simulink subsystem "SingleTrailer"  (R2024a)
settings: Solver=VariableStepAuto  StartTime=0.0  StopTime=10.0  RelTol=1e-3
undefined symbols (not defined in the file): D, PlntTraCGHgtAxl, PlntTraDstCGMiddleAxl, PlntTraHtchCxy, PlntTraHtchCz, PlntTraHtchF0z, PlntTraHtchKxy, PlntTraHtchKz, PlntTraInitLatPos, PlntTraInitLatVel, PlntTraInitLongPos, PlntTraInitLongVel, PlntTraInitPitchAng, PlntTraInitPitchRate, PlntTraInitRollAng, PlntTraInitRollRate, PlntTraInitVertPos, PlntTraInitVertVel, PlntTraInitYawAng, PlntTraInitYawRate, PlntTraMass, PlntTraNumWhlFrntAxl, PlntTraPitchMomentInertia, PlntTraRollMomentInertia, PlntTraTrckWdth, PlntTraYawMomentInertia, repmat, Row, vector
libraries: autolibutils x7, sharedtransform x4, vehdynlibeom x2, vehdynlibsuspension x1, matrix_library x1
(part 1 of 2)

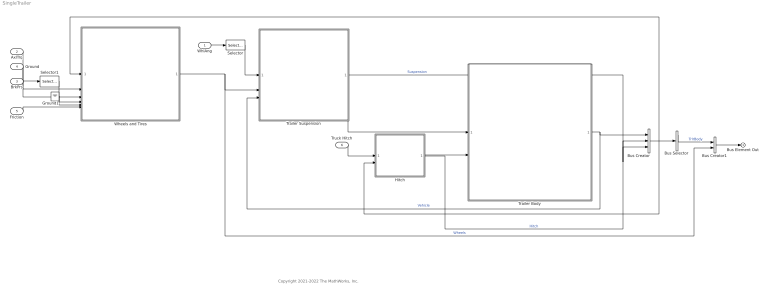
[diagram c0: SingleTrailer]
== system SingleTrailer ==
  note: Copyright 2021-2022 The MathWorks, Inc.
  WhlAng : Inport
  AxlTrq : Inport  Port=2
  BrkPrs : Inport  Port=3
  Ground : Inport  Port=4
  Friction : Inport  Port=5
  Truck Hitch : Inport  Port=6
  Bus Creator : BusCreator  Inputs=3
  Bus Creator1 : BusCreator  Inputs=2
  Bus Selector : BusSelector  OutputSignals=Vehicle.InertFrm,Vehicle.BdyFrm,Hitch,Suspension  OutputAsBus=on
  Ground1 : Ground
  Hitch : Subsystem  Variant=on  VariantControlMode=label  LabelModeActiveChoice=Hitch 3DOF
  Selector : Selector  IndexOptions=Index vector (dialog)  Indices=[1 2]  OutputSizes=1
  Selector1 : Selector  IndexOptions=Index vector (dialog)  Indices=[1 2]  OutputSizes=1
  Trailer Body : Subsystem  Variant=on  VariantControlMode=label  LabelModeActiveChoice=Trailer Body 3DOF
  Trailer Suspension : Subsystem
  Wheels and Tires : Subsystem  Variant=on  VariantControlMode=label  VariantControl=Choice  LabelModeActiveChoice=MF Tires Longitudinal and Lateral
  Bus Element Out : Outport
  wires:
  Trailer Suspension/1(SuspWheel) -> Bus Creator/2  "Suspension"
  Trailer Suspension/2(SuspChassis) -> Trailer Body/1(Suspension)
  Bus Selector/1 -> Bus Creator1/1  "TrlrBody"
  AxlTrq/1 -> Wheels and Tires/2(AxlTrq)
  Bus Creator/1 -> Bus Selector/1, Wheels and Tires/1(Suspension), Hitch/2(Trailer)
  Wheels and Tires/1(Wheels) -> Bus Creator1/2, Trailer Suspension/2(Wheels)  "Wheels"
  BrkPrs/1 -> Selector1/1
  WhlAng/1 -> Selector/1
  Friction/1 -> Wheels and Tires/6(Friction)
  Trailer Body/1(Vehicle) -> Bus Creator/1, Trailer Suspension/3(Veh)  "Vehicle"
  Truck Hitch/1 -> Hitch/1(Vehicle)
  Selector/1 -> Trailer Suspension/1(Steering)
  Selector1/1 -> Wheels and Tires/4(BrkPrs)
  Ground/1 -> Wheels and Tires/3(Ground Input)
  Ground1/1 -> Wheels and Tires/5(GndDCM)
  Hitch/1(Vehicle Hitch) -> Bus Creator/3  "Hitch"
  Hitch/2(Trailer Hitch) -> Trailer Body/2(Hitch)
  Bus Creator1/1 -> Bus Element Out/1

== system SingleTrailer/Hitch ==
  note: 1) Add Subsystem or Model blocks as valid variant choices. 2) You cannot connect blocks at this level. At simulation, connectivity is automatically determined, based on the active variant and port name matching.
  Vehicle : Inport
  Trailer : Inport  Port=2
  3DOF : Subsystem  VariantControl=Hitch 3DOF
  6DOF : Subsystem  VariantControl=Hitch 6DOF
  Vehicle Hitch : Outport
  Trailer Hitch : Outport  Port=2

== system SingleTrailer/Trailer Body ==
  note: 1) Add Subsystem or Model blocks as valid variant choices. 2) You cannot connect blocks at this level. At simulation, connectivity is automatically determined, based on the active variant and port name matching.
  Suspension : Inport
  Hitch : Inport  Port=2
  Trailer Body 3DOF : Subsystem  VariantControl=Trailer Body 3DOF
  Trailer Body 6DOF : Subsystem  VariantControl=Trailer Body 6DOF
  Vehicle : Outport

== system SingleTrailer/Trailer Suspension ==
  Steering : Inport
  Wheels : Inport  Port=2
  Veh : Inport  Port=3
  Bus Creator : BusCreator  Inputs=2
  Solid Axle Suspension : Subsystem  VariantControl=MacPherson Front Suspension Solid Axle Rear Suspension
  Susp2Wheel : Subsystem
  Wheel2Susp : Subsystem
  SuspWheel : Outport
  SuspChassis : Outport  Port=2
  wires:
  Steering/1 -> Solid Axle Suspension/1(Steer)
  Veh/1 -> Solid Axle Suspension/2(Vehicle), Wheel2Susp/1(Veh)
  Bus Creator/1 -> SuspChassis/1
  Wheels/1 -> Wheel2Susp/2(Wheels)
  Susp2Wheel/1(SuspWheel) -> Wheel2Susp/3(SuspWheel), Bus Creator/2, SuspWheel/1  "SuspWheel"
  Wheel2Susp/1(Wheels2Susp) -> Susp2Wheel/2(WheelSusp), Solid Axle Suspension/3(Wheels)
  Solid Axle Suspension/1(Suspension) -> Bus Creator/1, Susp2Wheel/1(Susp)  "SuspChassis"

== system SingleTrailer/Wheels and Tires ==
  Suspension : Inport
  AxlTrq : Inport  Port=2
  Ground Input : Inport  Port=3
  BrkPrs : Inport  Port=4
  GndDCM : Inport  Port=5
  Friction : Inport  Port=6
  Combined Slip Tires Longitudinal : Subsystem  VariantControl=Combined Slip Tires Longitudinal  ReferencedSubsystem=CombinedSlipTrailerTiresLongitudinal
  Fiala Tires Longitudinal and Lateral : Subsystem  VariantControl=Fiala Tires Longitudinal and Lateral  ReferencedSubsystem=FialaTrailerTires
  MF Tires Longitudinal : Subsystem  VariantControl=MF Tires Longitudinal  ReferencedSubsystem=MFTrailerTiresLongitudinal
  MF Tires Longitudinal and Lateral : Subsystem  VariantControl=MF Tires Longitudinal and Lateral  ReferencedSubsystem=MFTrailerTires
  Wheels : Outport

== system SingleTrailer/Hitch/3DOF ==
  Vehicle : Inport
  Trailer : Inport  Port=2
  Bus Selector : BusSelector  OutputSignals=Body.InertFrm.Hitch.Disp.X,Body.InertFrm.Hitch.Disp.Y,Body.InertFrm.Cg.Ang.psi,Body.InertFrm.Hitch.Vel.Xdot,Body.InertFrm.Hitch.Vel.Ydot
  Bus Selector1 : BusSelector  OutputSignals=Vehicle.InertFrm.HitchF.Disp.X,Vehicle.InertFrm.HitchF.Disp.Y,Vehicle.InertFrm.Cg.Ang.psi,Vehicle.BdyFrm.Forces.HitchF.Fz,Vehicle.InertFrm.HitchF.Vel.Xdot,Vehicle.InertFrm.HitchF.Vel.Ydot
  Mux : Mux  Inputs=6
  Mux1 : Mux  Inputs=6
  Subsystem3 : Subsystem
  Vehicle Hitch : Outport
  Trailer Hitch : Outport  Port=2
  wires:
  Subsystem3/9(Trailer FzOut) -> Mux/3
  Mux1/1 -> Vehicle Hitch/1
  Vehicle/1 -> Bus Selector/1
  Mux/1 -> Trailer Hitch/1
  Trailer/1 -> Bus Selector1/1
  Bus Selector/1 -> Subsystem3/1(Vehicle X)  "<X>"
  Bus Selector/2 -> Subsystem3/2(Vehicle Y)  "<Y>"
  Bus Selector/3 -> Subsystem3/3(Vehicle psi)  "<psi>"
  Bus Selector1/1 -> Subsystem3/6(Trailer X)  "<X>"
  Bus Selector1/2 -> Subsystem3/7(Trailer Y)  "<Y>"
  Bus Selector1/4 -> Subsystem3/9(Trailer Fz)  "<Fz>"
  Bus Selector1/3 -> Subsystem3/8(Trailer psi)  "<psi>"
  Subsystem3/1(Vehicle Fx) -> Mux1/1
  Subsystem3/2(Vehicle Fy) -> Mux1/2
  Subsystem3/3(Vehicle Fz) -> Mux1/3
  Subsystem3/7(Trailer Fx) -> Mux/1
  Subsystem3/8(Trailer Fy) -> Mux/2
  Bus Selector/4 -> Subsystem3/4(Vehicle Xdot)  "<Xdot>"
  Bus Selector/5 -> Subsystem3/5(Vehicle Ydot)  "<Ydot>"
  Bus Selector1/5 -> Subsystem3/10(Trailer Xdot)  "<Xdot>"
  Bus Selector1/6 -> Subsystem3/11(Trailer Ydot)  "<Ydot>"
  Subsystem3/10(Trailer Mhx) -> Mux/4
  Subsystem3/11(Trailer Mhy) -> Mux/5
  Subsystem3/12(Trailer Mhz) -> Mux/6
  Subsystem3/4(Vehicle Mhx) -> Mux1/4
  Subsystem3/5(Vehicle Mhy) -> Mux1/5
  Subsystem3/6(Vehicle Mhz) -> Mux1/6

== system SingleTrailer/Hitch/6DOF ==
  Vehicle : Inport
  Trailer : Inport  Port=2
  Bus Selector : BusSelector  OutputSignals=InertFrm.Hitch.Disp.X,InertFrm.Hitch.Disp.Y,InertFrm.Hitch.Disp.Z,InertFrm.Hitch.Vel.Xdot,InertFrm.Hitch.Vel.Ydot,InertFrm.Hitch.Vel.Zdot,InertFrm.Cg.Ang.psi
  Bus Selector1 : BusSelector  OutputSignals=Vehicle.InertFrm.HitchF.Disp.X,Vehicle.InertFrm.HitchF.Disp.Y,Vehicle.InertFrm.HitchF.Disp.Z,Vehicle.InertFrm.HitchF.Vel.Xdot,Vehicle.InertFrm.HitchF.Vel.Ydot,Vehicle.InertFrm.HitchF.Vel.Zdot,Vehicle.InertFrm.Cg.Ang.psi
  Mux : Mux  Inputs=6
  Mux1 : Mux  Inputs=6
  Subsystem3 : Subsystem
  Vehicle Hitch : Outport
  Trailer Hitch : Outport  Port=2
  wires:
  Subsystem3/9(Trailer Fz) -> Mux/3
  Mux1/1 -> Vehicle Hitch/1
  Vehicle/1 -> Bus Selector/1
  Mux/1 -> Trailer Hitch/1
  Trailer/1 -> Bus Selector1/1
  Bus Selector/1 -> Subsystem3/1(Vehicle X)  "<X>"
  Bus Selector/2 -> Subsystem3/2(Vehicle Y)  "<Y>"
  Bus Selector/7 -> Subsystem3/7(Vehicle psi)  "<psi>"
  Bus Selector1/1 -> Subsystem3/8(Trailer X)  "<X>"
  Bus Selector1/2 -> Subsystem3/9(Trailer Y)  "<Y>"
  Bus Selector1/7 -> Subsystem3/14(Trailer psi)  "<psi>"
  Subsystem3/1(Vehicle Fx) -> Mux1/1
  Subsystem3/2(Vehicle Fy) -> Mux1/2
  Subsystem3/3(Vehicle Fz) -> Mux1/3
  Subsystem3/7(Trailer Fx) -> Mux/1
  Subsystem3/8(Trailer Fy) -> Mux/2
  Bus Selector1/3 -> Subsystem3/10(Trailer Z)  "<Z>"
  Bus Selector/3 -> Subsystem3/3(Vehicle Z)  "<Z>"
  Bus Selector/6 -> Subsystem3/6(Vehicle Zdot)  "<Zdot>"
  Bus Selector1/6 -> Subsystem3/13(Trailer Zdot)  "<Zdot>"
  Bus Selector1/5 -> Subsystem3/12(Trailer Ydot)  "<Ydot>"
  Bus Selector1/4 -> Subsystem3/11(Trailer Xdot)  "<Xdot>"
  Bus Selector/4 -> Subsystem3/4(Vehicle Xdot)  "<Xdot>"
  Bus Selector/5 -> Subsystem3/5(Vehicle Ydot)  "<Ydot>"
  Subsystem3/10(Trailer Mhx) -> Mux/4
  Subsystem3/11(Trailer Mhy) -> Mux/5
  Subsystem3/12(Trailer Mhz) -> Mux/6
  Subsystem3/4(Vehicle Mhx) -> Mux1/4
  Subsystem3/5(Vehicle Mhy) -> Mux1/5
  Subsystem3/6(Vehicle Mhz) -> Mux1/6

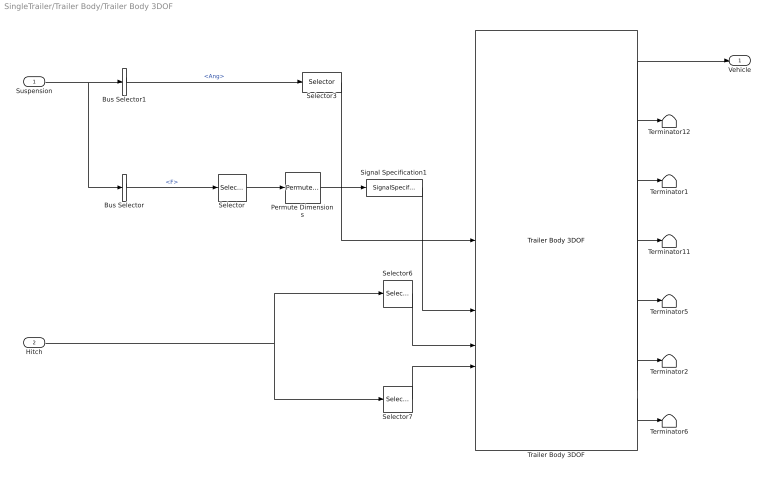
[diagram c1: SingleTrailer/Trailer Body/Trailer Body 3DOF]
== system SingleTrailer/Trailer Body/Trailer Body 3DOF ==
  Suspension : Inport
  Hitch : Inport  Port=2
  Bus Selector : BusSelector  OutputSignals=SuspChassis.Veh.F
  Bus Selector1 : BusSelector  OutputSignals=SuspChassis.Whl.Ang
  Permute Dimensions : PermuteDimensions
  Selector : Selector  NumberOfDimensions=2  InputPortWidth=3  IndexOptions=Index vector (dialog),Index vector (dialog)  Indices=[1 2],[1 2]  OutputSizes=1,1
  Selector3 : Selector  NumberOfDimensions=2  InputPortWidth=6  IndexOptions=Index vector (dialog),Index vector (dialog)  Indices=3,[1 2]  OutputSizes=1,1
  Selector6 : Selector  InputPortWidth=6  IndexOptions=Index vector (dialog)  Indices=[1 2 3]  OutputSizes=1
  Selector7 : Selector  InputPortWidth=6  IndexOptions=Index vector (dialog)  Indices=[4 5 6]  OutputSizes=1
  Signal Specification1 : SignalSpecification  Unit=N
  Terminator{1..2,5..6,11..12} (6 alike) : Terminator
  Trailer Body 3DOF : vehdynlibeom/Trailer Body 3DOF  trackMode=Dual 1-axle  inputMode=External forces  frontSteerMode=on  middleSteerMode=off  rearSteerMode=off  windMode=off  muMode=off  extFMode=off  extMMode=off  FhtchFMode=on  FhtchMMode=on  RhtchFMode=off  RhtchMMode=off  extXo=off  extpsio=off  extxdoto=off  extro=off  extYo=off  extTamb=off  extydoto=off  aMode=2  NF=PlntTraNumWhlFrntAxl  NM=PlntTraNumWhlMiddleAxl  NR=PlntTraNumWhlRearAxl  m=PlntTraMass  a=PlntTraDstCGFrntAxl  b=PlntTraDstCGMiddleAxl  c=PlntTraDstCGRearAxl  h=PlntTraCGHgtAxl  dh_f=PlntTraHtchDstFrnt  hh_f=PlntTraHtchHgtAxlFrnt  dh_r=7.5  hh_r=0.6  X_o=PlntTraInitLongPos  xdot_o=PlntTraInitLongVel  Lcpm=2.75  CalphaMode=off  sigmaMode=on  d=0  hl_f=0  hl_r=0  w_f=PlntTraTrckWdth  w_m=PlntTraTrckWdth  w_r=PlntTraTrckWdth  Cy_f=12e3  Cy_m=11e3  Cy_r=11e3  sigma_f=.1  sigma_m=.1  sigma_r=.1  alpha_f_brk=[-.1 .1]  Cy_f_data=[-9e3 9e3]  alpha_m_brk=[-.1 .1]  Cy_m_data=[-9e3 9e3]  alpha_r_brk=[-.1 .1]  Cy_r_data=[-9e3 9e3]  Y_o=PlntTraInitLatPos  ydot_o=PlntTraInitLatVel  Izz=PlntTraYawMomentInertia  psi_o=PlntTraInitYawAng  r_o=PlntTraInitYawRate  Af=PlntTraAeroFrntArea  Cd=PlntTraAeroDragCff  Cl=PlntTraAeroLiftCff  Cpm=PlntTraAeroPitchCff  beta_w=[0:0.01:0.3]  Cs=[0:0.03:0.9]*0  Cym=[0:0.01:0.3]*0  Pabs=101325  Tair=273  g=9.81  mu=1  xdot_tol=.01  Fznom=5000  Fxtire_sat=7e4  Fytire_sat=7e4  longOff=0  latOff=0  vertOff=0  wrapAng=off
  Vehicle : Outport
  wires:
  Suspension/1 -> Bus Selector/1, Bus Selector1/1
  Trailer Body 3DOF/6 -> Terminator2/1
  Trailer Body 3DOF/7 -> Terminator6/1
  Trailer Body 3DOF/2 -> Terminator12/1
  Trailer Body 3DOF/3 -> Terminator1/1
  Bus Selector1/1 -> Selector3/1  "<Ang>"
  Signal Specification1/1 -> Trailer Body 3DOF/2
  Selector3/1 -> Trailer Body 3DOF/1
  Trailer Body 3DOF/5 -> Terminator5/1
  Permute Dimensions/1 -> Signal Specification1/1
  Selector/1 -> Permute Dimensions/1
  Trailer Body 3DOF/1 -> Vehicle/1
  Bus Selector/1 -> Selector/1  "<F>"
  Trailer Body 3DOF/4 -> Terminator11/1
  Selector6/1 -> Trailer Body 3DOF/3
  Hitch/1 -> Selector7/1, Selector6/1
  Selector7/1 -> Trailer Body 3DOF/4

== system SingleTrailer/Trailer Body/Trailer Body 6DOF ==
  Suspension : Inport
  Hitch : Inport  Port=2
  Bus Selector3 : BusSelector  OutputSignals=SuspChassis.Veh.F,SuspChassis.Veh.M
  Constant1 : Constant  Value=zeros(3,1)  SampleTime=-1
  Constant2 : Constant  Value=zeros(3,1)  SampleTime=-1
  Constant3 : Constant  Value=zeros(3,1)  SampleTime=-1
  Selector6 : Selector  InputPortWidth=6  IndexOptions=Index vector (dialog)  Indices=[1 2 3]  OutputSizes=1
  Selector7 : Selector  InputPortWidth=6  IndexOptions=Index vector (dialog)  Indices=[4 5 6]  OutputSizes=1
  Terminator{,1..5} (6 alike) : Terminator
  Trailer Body 6DOF : vehdynlibeom/Trailer Body 6DOF  axleMode=1  extPos=on  extVel=on  extEuler=on  extRotRate=on  htchFMode_f=on  htchMMode_f=on  htchFMode_r=off  htchMMode_r=off  m=PlntTraMass  a=PlntTraDstCGFrntAxl  b=PlntTraDstCGMiddleAxl  c=PlntTraDstCGRearAxl  d=0  h=PlntTraCGHgtAxl  dh_f=PlntTraHtchDstFrnt  hl_f=0  hh_f=PlntTraHtchHgtAxlFrnt  dh_r=1  hl_r=0  hh_r=0.1  Xe_o=[PlntTraInitLongPos,PlntTraInitLatPos,PlntTraInitVertPos]  xbdot_o=[PlntTraInitLongVel,PlntTraInitLatVel,PlntTraInitVertVel]  eul_o=[PlntTraInitRollAng,PlntTraInitPitchAng,PlntTraInitYawAng]  p_o=[PlntTraInitRollRate,PlntTraInitPitchRate,PlntTraInitYawRate]  Iveh=[PlntTraRollMomentInertia 0 0; 0 PlntTraPitchMomentInertia 0; 0 0 PlntTraYawMomentInertia]  w_f=PlntTraTrckWdth  w_m=PlntTraTrckWdth  w_r=PlntTraTrckWdth  z1m=0  z1R=[-.25,.125,.15]  z1I=[1.4,-.2,.1;-.2,1.4,.1;.1,.1,2.25].*0  z2m=0  z2R=[1.4,0,.8]  z2I=[1.4,-.2,.1;-.2,1.4,.1;.1,.1,2.25].*0  z3m=0  z3R=[.75,-.5,.4]  z3I=[5,-.1,-2;-2,9,.1;-.1,.1,6].*0  z4m=0  z4R=[.75,.5,.4]  z4I=[5,-.1,-2;-2,9,.1;-.1,.1,6].*0  z5m=0  z5R=[1.25,-.5,.4]  z5I=[5,-.1,-2;-2,9,.1;-.1,.1,6].*0  z6m=0  z6R=[1.25,-.5,.4]  z6I=[5,-.1,-2;-2,9,.1;-.1,.1,6].*0  z7m=0  z7R=[2,0,.25]  z7I=[1.4,-.2,.1;-.2,1.4,.1;.1,.1,2.25].*0  Af=PlntTraAeroFrntArea  Cd=PlntTraAeroDragCff  Cl=PlntTraAeroLiftCff  Cpm=PlntTraAeroPitchCff  beta_w=[0:0.01:0.3]  Cs=[0:0.03:0.9]  Cym=[0:0.01:0.3]  Pabs=101325  extTamb=off  Tair=273  g=9.81  xdot_tol=.1  longOff=0  latOff=0  vertOff=0.0112  wrapAng=off  aMode=2
  Vehicle : Outport
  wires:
  Suspension/1 -> Bus Selector3/1
  Bus Selector3/2 -> Trailer Body 6DOF/2  "<M>"
  Bus Selector3/1 -> Trailer Body 6DOF/1  "<F>"
  Constant2/1 -> Trailer Body 6DOF/3
  Constant3/1 -> Trailer Body 6DOF/4
  Trailer Body 6DOF/7 -> Terminator/1
  Trailer Body 6DOF/6 -> Terminator1/1
  Trailer Body 6DOF/5 -> Terminator2/1
  Trailer Body 6DOF/4 -> Terminator3/1
  Trailer Body 6DOF/3 -> Terminator4/1
  Trailer Body 6DOF/2 -> Terminator5/1
  Trailer Body 6DOF/1 -> Vehicle/1
  Constant1/1 -> Trailer Body 6DOF/7
  Hitch/1 -> Selector7/1, Selector6/1
  Selector6/1 -> Trailer Body 6DOF/5
  Selector7/1 -> Trailer Body 6DOF/6

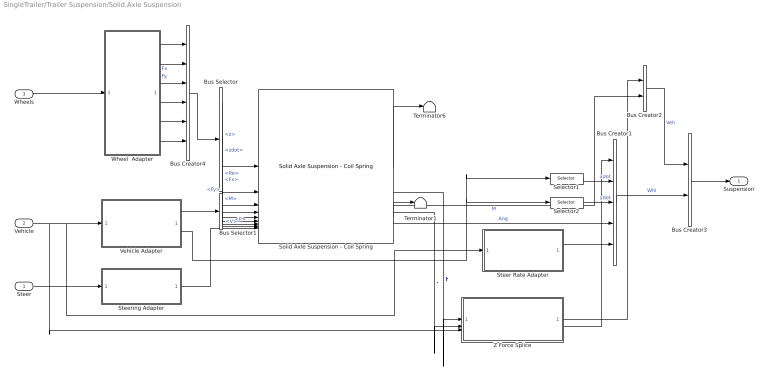
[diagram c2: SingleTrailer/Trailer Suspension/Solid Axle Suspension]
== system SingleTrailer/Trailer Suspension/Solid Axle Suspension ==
  Steer : Inport
  Vehicle : Inport  Port=2
  Wheels : Inport  Port=3
  Bus Creator1 : BusCreator  Inputs=5
  Bus Creator2 : BusCreator  Inputs=2
  Bus Creator3 : BusCreator  Inputs=2
  Bus Creator4 : BusCreator  Inputs=6
  Bus Selector : BusSelector  OutputSignals=z,Re,zdot,Fx,Fy,M
  Bus Selector1 : BusSelector  OutputSignals=P,V
  Selector1 : Selector  NumberOfDimensions=2  InputPortWidth=3  IndexOptions=Index vector (dialog),Select all  Indices=1,1  OutputSizes=1,1
  Selector2 : Selector  NumberOfDimensions=2  InputPortWidth=3  IndexOptions=Index vector (dialog),Select all  Indices=2,1  OutputSizes=1,1
  Solid Axle Suspension - Coil Spring : vehdynlibsuspension/Solid Axle Suspension - Coil Spring  NumAxl=1  NumWhlsByAxl=PlntTraNumWhlFrntAxl  StrgEnByAxl=1  WhlNumVec="[1  2]"  AxleNumVec="[1  1]"  SuspTypesByAxle=[1]  SuspImage=suspsacoil.png  AxlIxx=PlntTraAxlIxx  AxlM=PlntTraAxlM  TrackCoords=[zeros(1,2);PlntTraTrckWdth*[1 -1]/2;zeros(1,2)]  SuspCoords=[zeros(1,2);PlntTraTrckWdth*[1 -1]/2;zeros(1,2)]  KzWhlAxl=PlntTraKzWhlAxl  F0zWhlAxl=PlntTraF0zWhlAxl  CzWhlAxl=PlntTraCzWhlAxl  IdealSuspEn=on  IdealSuspAxles=[1]  Kz=PlntTraSuspKz  F0z=PlntTraSuspF0z  Cz=PlntTraSuspCz  Hmax=PlntTraSuspHmax  Toe=0  RollStrgSlp=0  ToeStrgSlp=0  Caster=0  CasterHslp=0  CasterStrgSlp=0  Camber=0  CamberHslp=0  CamberStrgSlp=0  StrgHgtSlp=0.1432  MappedSuspEn=off  MappedSuspAxles="[1  2]"  f_susp_axl_bp=[1 2]  f_susp_dz_bp=[-0.15 -0.14 -0.13 -0.12 -0.11 -0.10 -0.09 -0.08 -0.07 -0.06 -0.05 -0.04 -0.03 -0.02 -0.01 0.00 0.01 0.02 0.03 0.04 0.05 0.06 0.07 0.08 0.09 0.10 0.11 0.12 0.13 0.14 0.15]  f_susp_dzdot_bp=[-0.15 -0.14 -0.13 -0.12 -0.11 -0.10 -0.09 -0.08 -0.07 -0.06 -0.05 -0.04 -0.03 -0.02 -0.01 0.00 0.01 0.02 0.03 0.04 0.05 0.06 0.07 0.08 0.09 0.10 0.11 0.12 0.13 0.14 0.15]  f_susp_fmz=zeros(31,31,61,2,4)  f_susp_geom=zeros(31,61,2,3)  f_susp_strgdelta_bp=[-30,-29,-28,-27,-26,-25,-24,-23,-22,-21,-20,-19,-18,-17,-16,-15,-14,-13,-12,-11,-10,-9,-8,-7,-6,-5,-4,-3,-2,-1,0,1,2,3,4,5,6,7,8,9,10,11,12,13,14,15,16,17,18,19,20,21,22,23,24,25,26,27,28,29,30]
  Steer Rate Adapter : Subsystem
  Steering Adapter : Subsystem
  Terminator1 : Terminator
  Terminator6 : Terminator
  Vehicle Adapter : Subsystem
  Wheel  Adapter : Subsystem
  Z Force Splice : Subsystem  Variant=on  VariantControlMode=label  LabelModeActiveChoice=0
  Suspension : Outport
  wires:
  Steer/1 -> Steering Adapter/1(Steer)
  Wheels/1 -> Wheel  Adapter/1(Wheels)
  Bus Selector/6 -> Solid Axle Suspension - Coil Spring/6  "<M>"
  Wheel  Adapter/4(zdot) -> Bus Creator4/4
  Bus Creator2/1 -> Bus Creator3/1  "Veh"
  Bus Creator4/1 -> Bus Selector/1
  Wheel  Adapter/6(Re) -> Bus Creator4/6
  Bus Creator3/1 -> Suspension/1
  Bus Selector/3 -> Solid Axle Suspension - Coil Spring/3  "<zdot>"
  Solid Axle Suspension - Coil Spring/5 -> Terminator1/1
  Z Force Splice/2(WhlF) -> Bus Creator1/1
  Selector2/1 -> Bus Creator1/3  "ydot"
  Steer Rate Adapter/1(AngVel) -> Bus Creator1/5
  Solid Axle Suspension - Coil Spring/1 -> Terminator6/1
  Solid Axle Suspension - Coil Spring/4 -> Z Force Splice/2(WhlFIn)  "F"
  Solid Axle Suspension - Coil Spring/6 -> Bus Creator1/4  "Ang"
  Bus Creator1/1 -> Bus Creator3/2  "Whl"
  Bus Selector/1 -> Solid Axle Suspension - Coil Spring/1  "<z>"
  Bus Selector/4 -> Solid Axle Suspension - Coil Spring/4  "<Fx>"
  Steering Adapter/1(StrgAng) -> Solid Axle Suspension - Coil Spring/9
  Wheel  Adapter/3(z) -> Bus Creator4/3
  Bus Selector1/1 -> Solid Axle Suspension - Coil Spring/7  "<P>"
  Solid Axle Suspension - Coil Spring/2 -> Z Force Splice/1(VehFIn)  "F"
  Selector1/1 -> Bus Creator1/2  "xdot"
  Bus Selector1/2 -> Solid Axle Suspension - Coil Spring/8  "<V>"
  Wheel  Adapter/5(M) -> Bus Creator4/5
  Bus Selector/2 -> Solid Axle Suspension - Coil Spring/2  "<Re>"
  Vehicle Adapter/2(VehVbody) -> Selector2/1, Selector1/1
  Wheel  Adapter/1(WhlFx) -> Bus Creator4/1  "Fx"
  Vehicle Adapter/1(VehSusp) -> Bus Selector1/1
  Z Force Splice/1(VehF) -> Bus Creator2/1
  Solid Axle Suspension - Coil Spring/3 -> Bus Creator2/2  "M"
  Wheel  Adapter/2(WhlFy) -> Bus Creator4/2  "Fy"
  Vehicle/1 -> Vehicle Adapter/1(Veh), Steer Rate Adapter/1(Veh), Z Force Splice/3(Vehicle)
  Bus Selector/5 -> Solid Axle Suspension - Coil Spring/5  "<Fy>"

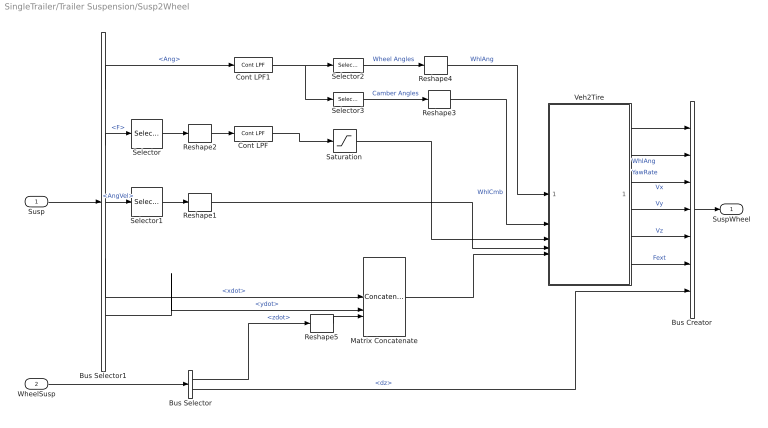
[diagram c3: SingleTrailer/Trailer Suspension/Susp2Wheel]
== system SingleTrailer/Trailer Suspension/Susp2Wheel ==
  Susp : Inport
  WheelSusp : Inport  Port=2
  Bus Creator : BusCreator  Inputs=7
  Bus Selector : BusSelector  OutputSignals=SuspFrame.zdot,SuspFrame.dz
  Bus Selector1 : BusSelector  OutputSignals=Whl.Ang,Whl.F,Whl.AngVel,Whl.xdot,Whl.ydot
  Cont LPF : autolibutils/Cont LPF  wc=100*2*pi  AbsoluteTolerance=auto  aMode=2
  Cont LPF1 : autolibutils/Cont LPF  wc=100*2*pi  AbsoluteTolerance=auto  aMode=2
  Matrix Concatenate : Concatenate  NumInputs=3  Mode=Multidimensional array
  Reshape{1..4} (4 alike) : Reshape
  Reshape5 : Reshape  OutputDimensionality=Row vector (2-D)
  Saturation : Saturate  UpperLimit=inf  LowerLimit=-10*9.81*2000  ZeroCross=off
  Selector : Selector  NumberOfDimensions=2  InputPortWidth=3  IndexOptions=Index vector (dialog),Select all  Indices=[3],1  OutputSizes=1,1
  Selector1 : Selector  NumberOfDimensions=2  InputPortWidth=1  IndexOptions=Index vector (dialog),Select all  Indices=[3],1  OutputSizes=1,1
  Selector2 : Selector  NumberOfDimensions=2  InputPortWidth=3  IndexOptions=Index vector (dialog),Select all  Indices=3,1  OutputSizes=1,1
  Selector3 : Selector  NumberOfDimensions=2  InputPortWidth=3  IndexOptions=Index vector (dialog),Select all  Indices=1,1  OutputSizes=1,1
  Veh2Tire : Subsystem
  SuspWheel : Outport
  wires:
  Bus Selector/2 -> Bus Creator/7  "<dz>"
  Veh2Tire/2(YawRate) -> Bus Creator/2  "YawRate"
  Bus Selector1/2 -> Selector/1  "<F>"
  Cont LPF1/1 -> Selector2/1, Selector3/1
  Reshape1/1 -> Veh2Tire/4(r)
  Selector2/1 -> Reshape4/1  "Wheel Angles"
  Reshape2/1 -> Cont LPF/1
  Selector3/1 -> Reshape3/1  "Camber Angles"
  Reshape3/1 -> Veh2Tire/2(SteerCmb)  "WhlCmb"
  Veh2Tire/1(WhlAng) -> Bus Creator/1  "WhlAng"
  Reshape4/1 -> Veh2Tire/1(SteerAng)  "WhlAng"
  Bus Selector1/4 -> Matrix Concatenate/1  "<xdot>"
  Bus Selector1/3 -> Selector1/1  "<AngVel>"
  Bus Selector1/5 -> Matrix Concatenate/2  "<ydot>"
  Veh2Tire/6(Fext) -> Bus Creator/6  "Fext"
  Selector1/1 -> Reshape1/1
  Saturation/1 -> Veh2Tire/3(Fz)
  Matrix Concatenate/1 -> Veh2Tire/5(VehVel)
  Selector/1 -> Reshape2/1
  Cont LPF/1 -> Saturation/1
  WheelSusp/1 -> Bus Selector/1
  Reshape5/1 -> Matrix Concatenate/3
  Bus Selector1/1 -> Cont LPF1/1  "<Ang>"
  Veh2Tire/5(Vz) -> Bus Creator/5  "Vz"
  Susp/1 -> Bus Selector1/1
  Veh2Tire/4(Vy) -> Bus Creator/4  "Vy"
  Veh2Tire/3(Vx) -> Bus Creator/3  "Vx"
  Bus Selector/1 -> Reshape5/1  "<zdot>"
  Bus Creator/1 -> SuspWheel/1

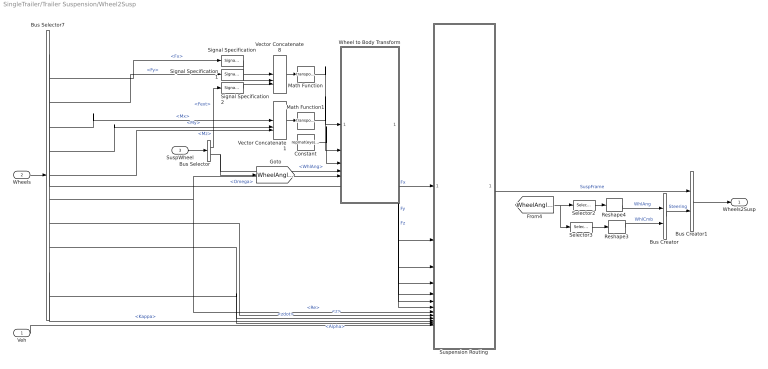
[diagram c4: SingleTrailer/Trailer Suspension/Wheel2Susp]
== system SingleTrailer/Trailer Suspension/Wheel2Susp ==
  Veh : Inport
  Wheels : Inport  Port=2
  SuspWheel : Inport  Port=3
  Bus Creator : BusCreator  Inputs=2
  Bus Creator1 : BusCreator  Inputs=2
  Bus Selector : BusSelector  OutputSignals=Fext,WhlAng
  Bus Selector7 : BusSelector  OutputSignals=Wheels.TireFrame.Omega,Wheels.TireFrame.Fx,Wheels.TireFrame.Fy,Wheels.TireFrame.Mx,Wheels.TireFrame.My,Wheels.TireFrame.Mz,Wheels.TireFrame.Re,Wheels.TireFrame.z,Wheels.TireFrame.zdot,Wheels.TireFrame.Kappa,Wheels.TireFrame.Alpha
  Constant : Constant  Value=repmat(eye(3),[1,1,2])
  Math Function : Math  Operator=transpose  SignedPower=on
  Math Function1 : Math  Operator=transpose  SignedPower=on
  Reshape3 : Reshape
  Reshape4 : Reshape
  Selector2 : Selector  NumberOfDimensions=2  InputPortWidth=3  IndexOptions=Index vector (dialog),Select all  Indices=3,1  OutputSizes=1,1
  Selector3 : Selector  NumberOfDimensions=2  InputPortWidth=3  IndexOptions=Index vector (dialog),Select all  Indices=1,1  OutputSizes=1,1
  Signal Specification : SignalSpecification  Dimensions=2
  Signal Specification1 : SignalSpecification  Dimensions=2
  Signal Specification2 : SignalSpecification  Dimensions=2
  Suspension Routing : Subsystem
  Vector Concatenate1 : Concatenate  NumInputs=3  Mode=Multidimensional array  ConcatenateDimension=2
  Vector Concatenate8 : Concatenate  NumInputs=3  Mode=Multidimensional array  ConcatenateDimension=2
  Wheel to Body Transform : Subsystem
  Wheels2Susp : Outport  VectorParamsAs1DForOutWhenUnconnected=off
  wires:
  Signal Specification1/1 -> Vector Concatenate8/2
  Signal Specification/1 -> Vector Concatenate8/1
  Veh/1 -> Suspension Routing/13(Veh)
  Bus Creator/1 -> Bus Creator1/2  "Steering"
  Reshape3/1 -> Bus Creator/2  "WhlCmb"
  Suspension Routing/1(SuspFrame) -> Bus Creator1/1  "SuspFrame"
  Bus Creator1/1 -> Wheels2Susp/1
  Reshape4/1 -> Bus Creator/1  "WhlAng"
  Wheel to Body Transform/3(Fz) -> Suspension Routing/4(Fz)  "Fz"
  Bus Selector/2 -> [WheelAngles], Wheel to Body Transform/4(WheelAngles)  "<WhlAng>"
  Wheels/1 -> Bus Selector7/1
  Math Function/1 -> Wheel to Body Transform/1(Forces)
  Vector Concatenate8/1 -> Math Function/1
  Wheel to Body Transform/1(Fx) -> Suspension Routing/2(Fx)  "Fx"
  Wheel to Body Transform/2(Fy) -> Suspension Routing/3(Fy)  "Fy"
  SuspWheel/1 -> Bus Selector/1
  Bus Selector/1 -> Signal Specification2/1  "<Fext>"
  Signal Specification2/1 -> Vector Concatenate8/3
  Selector2/1 -> Reshape4/1
  [WheelAngles] -> Selector2/1, Selector3/1
  Selector3/1 -> Reshape3/1
  Wheel to Body Transform/4(Mx) -> Suspension Routing/5(<Mx>)
  Wheel to Body Transform/5(My) -> Suspension Routing/6(<My>)
  Wheel to Body Transform/6(Mz) -> Suspension Routing/7(<Mz>)
  Vector Concatenate1/1 -> Math Function1/1
  Math Function1/1 -> Wheel to Body Transform/2(Moments)
  Constant/1 -> Wheel to Body Transform/3(DCM)
  Bus Selector7/1 -> Suspension Routing/1(Omega)  "<Omega>"
  Bus Selector7/2 -> Signal Specification/1  "<Fx>"
  Bus Selector7/3 -> Signal Specification1/1  "<Fy>"
  Bus Selector7/4 -> Vector Concatenate1/1  "<Mx>"
  Bus Selector7/5 -> Vector Concatenate1/2  "<My>"
  Bus Selector7/6 -> Vector Concatenate1/3  "<Mz>"
  Bus Selector7/7 -> Wheel to Body Transform/5(Re), Suspension Routing/8(<Re>)  "<Re>"
  Bus Selector7/8 -> Suspension Routing/9(<z>)  "<z>"
  Bus Selector7/9 -> Suspension Routing/10(<zdot>)  "<zdot>"
  Bus Selector7/10 -> Suspension Routing/11(<Kappa>)  "<Kappa>"
  Bus Selector7/11 -> Suspension Routing/12(<Alpha>)  "<Alpha>"

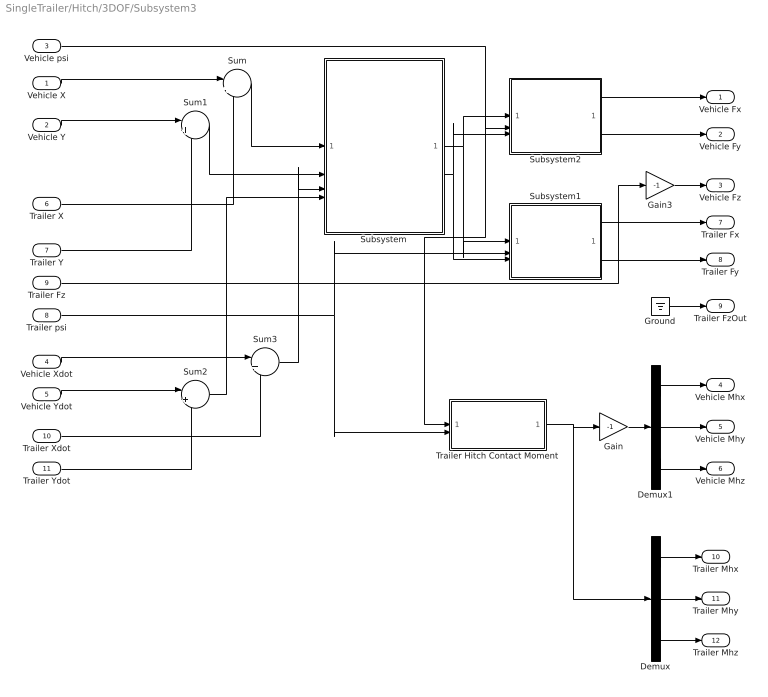
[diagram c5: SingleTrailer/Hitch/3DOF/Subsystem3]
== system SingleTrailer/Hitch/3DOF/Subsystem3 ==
  Vehicle X : Inport
  Vehicle Y : Inport  Port=2
  Vehicle psi : Inport  Port=3
  Vehicle Xdot : Inport  Port=4
  Vehicle Ydot : Inport  Port=5
  Trailer X : Inport  Port=6
  Trailer Y : Inport  Port=7
  Trailer psi : Inport  Port=8
  Trailer Fz : Inport  Port=9
  Trailer Xdot : Inport  Port=10
  Trailer Ydot : Inport  Port=11
  Demux : Demux  Outputs=3
  Demux1 : Demux  Outputs=3
  Gain : Gain  Gain=-1
  Gain3 : Gain  Gain=-1
  Ground : Ground
  Subsystem : Subsystem
  Subsystem1 : Subsystem
  Subsystem2 : Subsystem
  Sum{,1..3} (4 alike) : Sum  Inputs=|+-
  Trailer Hitch Contact Moment : Subsystem
  Vehicle Fx : Outport
  Vehicle Fy : Outport  Port=2
  Vehicle Fz : Outport  Port=3
  Vehicle Mhx : Outport  Port=4
  Vehicle Mhy : Outport  Port=5
  Vehicle Mhz : Outport  Port=6
  Trailer Fx : Outport  Port=7
  Trailer Fy : Outport  Port=8
  Trailer FzOut : Outport  Port=9
  Trailer Mhx : Outport  Port=10
  Trailer Mhy : Outport  Port=11
  Trailer Mhz : Outport  Port=12
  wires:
  Trailer Fz/1 -> Gain3/1
  Subsystem/2(Hitch Angles) -> Subsystem2/3(Hitch Angles), Subsystem1/3(Hitch Angles)
  Vehicle psi/1 -> Trailer Hitch Contact Moment/1(Vehicle Psi), Subsystem2/2(psi)
  Trailer psi/1 -> Subsystem1/2(psi), Trailer Hitch Contact Moment/2(Trailer Psi)
  Subsystem2/2(Fy) -> Vehicle Fy/1
  Subsystem2/1(Fx) -> Vehicle Fx/1
  Vehicle Y/1 -> Sum1/1
  Trailer Y/1 -> Sum1/2
  Subsystem1/2(Fy) -> Trailer Fy/1
  Gain3/1 -> Vehicle Fz/1
  Sum1/1 -> Subsystem/2(delta Y)
  Subsystem1/1(Fx) -> Trailer Fx/1
  Sum/1 -> Subsystem/1(delta X)
  Subsystem/1(Hitch Forces) -> Subsystem2/1(Hitch Forces), Subsystem1/1(Hitch Forces)
  Vehicle X/1 -> Sum/1
  Trailer X/1 -> Sum/2
  Trailer Xdot/1 -> Sum3/2
  Trailer Ydot/1 -> Sum2/2
  Vehicle Xdot/1 -> Sum3/1
  Vehicle Ydot/1 -> Sum2/1
  Sum3/1 -> Subsystem/3(delta Xdot)
  Sum2/1 -> Subsystem/4(delta Ydot)
  Demux1/2 -> Vehicle Mhy/1
  Demux1/1 -> Vehicle Mhx/1
  Demux/1 -> Trailer Mhx/1
  Demux1/3 -> Vehicle Mhz/1
  Demux/3 -> Trailer Mhz/1
  Trailer Hitch Contact Moment/1(Mh) -> Demux/1, Gain/1
  Gain/1 -> Demux1/1
  Demux/2 -> Trailer Mhy/1
  Ground/1 -> Trailer FzOut/1

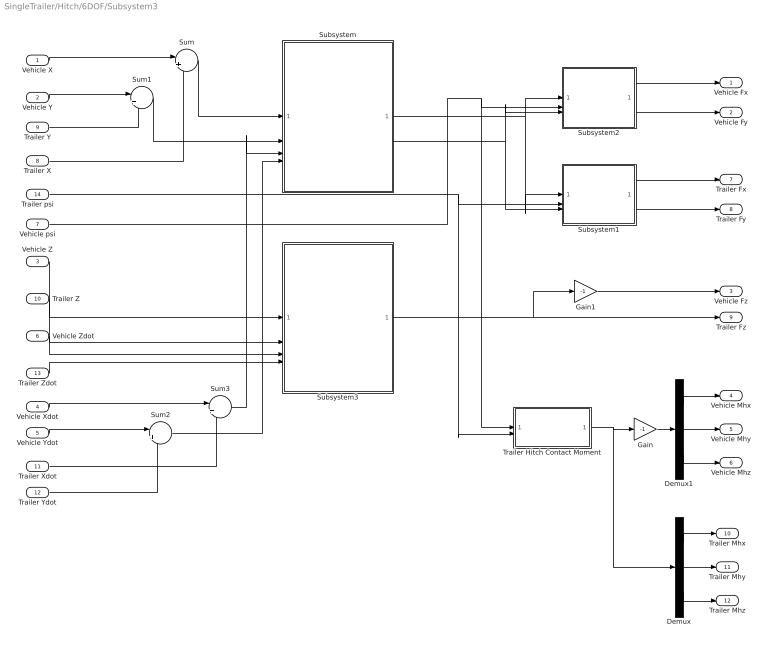
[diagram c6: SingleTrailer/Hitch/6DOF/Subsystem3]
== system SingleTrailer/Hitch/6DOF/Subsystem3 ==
  Vehicle X : Inport
  Vehicle Y : Inport  Port=2
  Vehicle Z : Inport  Port=3
  Vehicle Xdot : Inport  Port=4
  Vehicle Ydot : Inport  Port=5
  Vehicle Zdot : Inport  Port=6
  Vehicle psi : Inport  Port=7
  Trailer X : Inport  Port=8
  Trailer Y : Inport  Port=9
  Trailer Z : Inport  Port=10
  Trailer Xdot : Inport  Port=11
  Trailer Ydot : Inport  Port=12
  Trailer Zdot : Inport  Port=13
  Trailer psi : Inport  Port=14
  Demux : Demux  Outputs=3
  Demux1 : Demux  Outputs=3
  Gain : Gain  Gain=-1
  Gain1 : Gain  Gain=-1
  Subsystem : Subsystem
  Subsystem1 : Subsystem
  Subsystem2 : Subsystem
  Subsystem3 : Subsystem
  Sum{,1..3} (4 alike) : Sum  Inputs=|+-
  Trailer Hitch Contact Moment : Subsystem
  Vehicle Fx : Outport
  Vehicle Fy : Outport  Port=2
  Vehicle Fz : Outport  Port=3
  Vehicle Mhx : Outport  Port=4
  Vehicle Mhy : Outport  Port=5
  Vehicle Mhz : Outport  Port=6
  Trailer Fx : Outport  Port=7
  Trailer Fy : Outport  Port=8
  Trailer Fz : Outport  Port=9
  Trailer Mhx : Outport  Port=10
  Trailer Mhy : Outport  Port=11
  Trailer Mhz : Outport  Port=12
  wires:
  Subsystem/1(Hitch Forces) -> Subsystem2/1(Hitch Forces), Subsystem1/1(Hitch Forces)
  Sum/1 -> Subsystem/1(delta X)
  Sum1/1 -> Subsystem/2(delta Y)
  Vehicle X/1 -> Sum/1
  Trailer Y/1 -> Sum1/2
  Trailer X/1 -> Sum/2
  Vehicle Y/1 -> Sum1/1
  Trailer psi/1 -> Subsystem1/2(psi), Trailer Hitch Contact Moment/2(Trailer Psi)
  Vehicle psi/1 -> Subsystem2/2(psi), Trailer Hitch Contact Moment/1(Vehicle Psi)
  Subsystem/2(Hitch Angles) -> Subsystem2/3(Hitch Angles), Subsystem1/3(Hitch Angles)
  Subsystem3/1(Trailer Fz) -> Gain1/1, Trailer Fz/1
  Subsystem2/1(Fx) -> Vehicle Fx/1
  Subsystem2/2(Fy) -> Vehicle Fy/1
  Subsystem1/1(Fx) -> Trailer Fx/1
  Subsystem1/2(Fy) -> Trailer Fy/1
  Vehicle Z/1 -> Subsystem3/1(Vehicle Z)
  Trailer Z/1 -> Subsystem3/2(Trailer Z)
  Gain1/1 -> Vehicle Fz/1
  Vehicle Zdot/1 -> Subsystem3/3(Vehicle Zdot)
  Trailer Zdot/1 -> Subsystem3/4(Trailer Zdot)
  Trailer Ydot/1 -> Sum2/2
  Vehicle Xdot/1 -> Sum3/1
  Vehicle Ydot/1 -> Sum2/1
  Trailer Xdot/1 -> Sum3/2
  Sum2/1 -> Subsystem/4(delta Ydot)
  Sum3/1 -> Subsystem/3(delta Xdot)
  Demux1/3 -> Vehicle Mhz/1
  Trailer Hitch Contact Moment/1(Mh) -> Demux/1, Gain/1
  Demux/1 -> Trailer Mhx/1
  Demux1/2 -> Vehicle Mhy/1
  Demux/2 -> Trailer Mhy/1
  Demux1/1 -> Vehicle Mhx/1
  Gain/1 -> Demux1/1
  Demux/3 -> Trailer Mhz/1

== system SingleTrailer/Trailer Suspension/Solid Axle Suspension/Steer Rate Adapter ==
  Veh : Inport
  Add : Sum
  Bus Selector3 : BusSelector  OutputSignals=BdyFrm.Cg.AngVel.r
  Constant : Constant  Value=zeros(1,2)  SampleTime=-1
  Matrix Concatenate : Concatenate  NumInputs=3  Mode=Multidimensional array
  Matrix Concatenate1 : Concatenate  NumInputs=3  Mode=Multidimensional array
  Mux : Mux  Inputs=2
  Reshape2 : Reshape  OutputDimensionality=Row vector (2-D)
  Reshape3 : Reshape  OutputDimensionality=Row vector (2-D)
  Reshape4 : Reshape  OutputDimensionality=Row vector (2-D)
  SteerRates : Constant  Value=zeros(1,2)  SampleTime=-1
  AngVel : Outport  VectorParamsAs1DForOutWhenUnconnected=off
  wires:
  Add/1 -> AngVel/1  "AngVel"
  Veh/1 -> Bus Selector3/1
  Matrix Concatenate1/1 -> Add/1
  Reshape3/1 -> Matrix Concatenate/1, Matrix Concatenate/2
  Reshape4/1 -> Matrix Concatenate/3
  SteerRates/1 -> Reshape2/1
  Matrix Concatenate/1 -> Add/2
  Bus Selector3/1 -> Mux/1, Mux/2  "<r>"
  Mux/1 -> Reshape4/1
  Constant/1 -> Reshape3/1
  Reshape2/1 -> Matrix Concatenate1/2, Matrix Concatenate1/3, Matrix Concatenate1/1

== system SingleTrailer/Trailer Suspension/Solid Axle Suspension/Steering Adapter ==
  Steer : Inport
  Reshape1 : Reshape  OutputDimensionality=Row vector (2-D)
  StrgAng : Outport  VectorParamsAs1DForOutWhenUnconnected=off
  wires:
  Steer/1 -> Reshape1/1
  Reshape1/1 -> StrgAng/1

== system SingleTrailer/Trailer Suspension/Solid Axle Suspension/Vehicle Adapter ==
  Veh : Inport
  Bus Creator3 : BusCreator  Inputs=2
  Bus Selector1 : BusSelector  OutputSignals=InertFrm.FrntAxl.Lft.Disp.X,InertFrm.FrntAxl.Lft.Disp.Y,InertFrm.FrntAxl.Lft.Disp.Z,InertFrm.FrntAxl.Rght.Disp.X,InertFrm.FrntAxl.Rght.Disp.Y,InertFrm.FrntAxl.Rght.Disp.Z
  Bus Selector2 : BusSelector  OutputSignals=BdyFrm.FrntAxl.Lft.Vel.xdot,BdyFrm.FrntAxl.Lft.Vel.ydot,BdyFrm.FrntAxl.Lft.Vel.zdot,BdyFrm.FrntAxl.Rght.Vel.xdot,BdyFrm.FrntAxl.Rght.Vel.ydot,BdyFrm.FrntAxl.Rght.Vel.zdot
  Bus Selector3 : BusSelector  OutputSignals=InertFrm.FrntAxl.Lft.Vel.Xdot,InertFrm.FrntAxl.Lft.Vel.Ydot,InertFrm.FrntAxl.Lft.Vel.Zdot,InertFrm.FrntAxl.Rght.Vel.Xdot,InertFrm.FrntAxl.Rght.Vel.Ydot,InertFrm.FrntAxl.Rght.Vel.Zdot
  Inertial Frame CG to Axle Offset : Constant  Value=[zeros(2,2);PlntTraCGHgtAxl*ones(1,2)]  SampleTime=-1
  Mux1 : Mux  Inputs=6
  Mux2 : Mux  Inputs=6
  Mux3 : Mux  Inputs=6
  Reshape : Reshape  OutputDimensionality=Customize  OutputDimensions=[3,2]
  Reshape1 : Reshape  OutputDimensionality=Customize  OutputDimensions=[3,2]
  Reshape2 : Reshape  OutputDimensionality=Customize  OutputDimensions=[3,2]
  Sum : Sum  Inputs=|+-
  VehSusp : Outport  VectorParamsAs1DForOutWhenUnconnected=off
  VehVbody : Outport  Port=2  VectorParamsAs1DForOutWhenUnconnected=off
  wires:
  Veh/1 -> Bus Selector3/1, Bus Selector2/1, Bus Selector1/1
  Reshape2/1 -> VehVbody/1  "V"
  Bus Creator3/1 -> VehSusp/1  "Veh"
  Reshape/1 -> Sum/1
  Mux1/1 -> Reshape2/1
  Mux2/1 -> Reshape/1
  Inertial Frame CG to Axle Offset/1 -> Sum/2
  Sum/1 -> Bus Creator3/1  "P"
  Mux3/1 -> Reshape1/1
  Reshape1/1 -> Bus Creator3/2  "V"
  Bus Selector1/3 -> Mux2/3  "<Z>"
  Bus Selector1/2 -> Mux2/2  "<Y>"
  Bus Selector1/4 -> Mux2/4  "<X>"
  Bus Selector1/1 -> Mux2/1  "<X>"
  Bus Selector1/5 -> Mux2/5  "<Y>"
  Bus Selector1/6 -> Mux2/6  "<Z>"
  Bus Selector3/1 -> Mux3/1  "<Xdot>"
  Bus Selector3/2 -> Mux3/2  "<Ydot>"
  Bus Selector3/3 -> Mux3/3  "<Zdot>"
  Bus Selector3/4 -> Mux3/4  "<Xdot>"
  Bus Selector3/5 -> Mux3/5  "<Ydot>"
  Bus Selector3/6 -> Mux3/6  "<Zdot>"
  Bus Selector2/1 -> Mux1/1  "<xdot>"
  Bus Selector2/2 -> Mux1/2  "<ydot>"
  Bus Selector2/3 -> Mux1/3  "<zdot>"
  Bus Selector2/4 -> Mux1/4  "<xdot>"
  Bus Selector2/5 -> Mux1/5  "<ydot>"
  Bus Selector2/6 -> Mux1/6  "<zdot>"

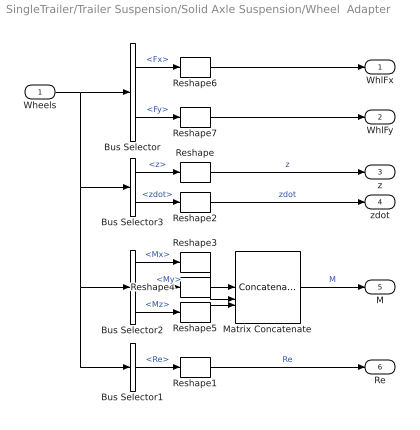
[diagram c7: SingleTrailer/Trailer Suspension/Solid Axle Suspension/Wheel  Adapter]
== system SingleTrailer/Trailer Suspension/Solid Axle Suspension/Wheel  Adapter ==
  Wheels : Inport
  Bus Selector : BusSelector  OutputSignals=SuspFrame.Fx,SuspFrame.Fy
  Bus Selector1 : BusSelector  OutputSignals=SuspFrame.Re
  Bus Selector2 : BusSelector  OutputSignals=SuspFrame.Mx,SuspFrame.My,SuspFrame.Mz
  Bus Selector3 : BusSelector  OutputSignals=SuspFrame.z,SuspFrame.zdot
  Matrix Concatenate : Concatenate  NumInputs=3  Mode=Multidimensional array
  Reshape{,1..7} (8 alike) : Reshape  OutputDimensionality=Row vector (2-D)
  WhlFx : Outport  VectorParamsAs1DForOutWhenUnconnected=off
  WhlFy : Outport  Port=2  VectorParamsAs1DForOutWhenUnconnected=off
  z : Outport  Port=3  VectorParamsAs1DForOutWhenUnconnected=off
  zdot : Outport  Port=4  VectorParamsAs1DForOutWhenUnconnected=off
  M : Outport  Port=5  VectorParamsAs1DForOutWhenUnconnected=off
  Re : Outport  Port=6  VectorParamsAs1DForOutWhenUnconnected=off
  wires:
  Reshape/1 -> z/1  "z"
  Matrix Concatenate/1 -> M/1  "M"
  Reshape5/1 -> Matrix Concatenate/3
  Reshape4/1 -> Matrix Concatenate/2
  Reshape3/1 -> Matrix Concatenate/1
  Bus Selector2/3 -> Reshape5/1  "<Mz>"
  Bus Selector2/2 -> Reshape4/1  "<My>"
  Bus Selector2/1 -> Reshape3/1  "<Mx>"
  Reshape1/1 -> Re/1  "Re"
  Bus Selector1/1 -> Reshape1/1  "<Re>"
  Reshape2/1 -> zdot/1  "zdot"
  Bus Selector3/2 -> Reshape2/1  "<zdot>"
  Wheels/1 -> Bus Selector/1, Bus Selector3/1, Bus Selector2/1, Bus Selector1/1
  Bus Selector3/1 -> Reshape/1  "<z>"
  Bus Selector/2 -> Reshape7/1  "<Fy>"
  Bus Selector/1 -> Reshape6/1  "<Fx>"
  Reshape6/1 -> WhlFx/1
  Reshape7/1 -> WhlFy/1

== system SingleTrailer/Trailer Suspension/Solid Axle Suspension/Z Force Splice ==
  note: 1) Add Subsystem or Model blocks as valid variant choices. 2) You cannot connect blocks at this level. At simulation, connectivity is automatically determined, based on the active variant and port name matching.
  VehFIn : Inport
  WhlFIn : Inport  Port=2
  Vehicle : Inport  Port=3
  Z Force Pass Through 6DOF : Subsystem  VariantControl=1
  Z Force Splice 3DOF : Subsystem  VariantControl=0
  VehF : Outport
  WhlF : Outport  Port=2

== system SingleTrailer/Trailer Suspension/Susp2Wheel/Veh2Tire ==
  SteerAng : Inport
  SteerCmb : Inport  Port=2
  Fz : Inport  Port=3
  r : Inport  Port=4
  VehVel : Inport  Port=5
  Reshape1 : Reshape
  Reshape2 : Reshape
  Reshape5 : Reshape
  Unary Minus : UnaryMinus
  Wheel Angles : Subsystem
  Wheel to Body Transform : Subsystem
  WhlAng : Outport  Unit=rad  VectorParamsAs1DForOutWhenUnconnected=off
  YawRate : Outport  Port=2  Unit=rad/s  VectorParamsAs1DForOutWhenUnconnected=off
  Vx : Outport  Port=3  Unit=m/s  VectorParamsAs1DForOutWhenUnconnected=off
  Vy : Outport  Port=4  Unit=m/s  VectorParamsAs1DForOutWhenUnconnected=off
  Vz : Outport  Port=5  Unit=m/s  VectorParamsAs1DForOutWhenUnconnected=off
  Fext : Outport  Port=6  Unit=N  VectorParamsAs1DForOutWhenUnconnected=off
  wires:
  SteerCmb/1 -> Wheel Angles/2(SteerCmb)
  Reshape5/1 -> Vz/1
  Reshape2/1 -> Vy/1
  Reshape1/1 -> Vx/1
  Wheel Angles/1("WhlAng ") -> Wheel to Body Transform/2(WheelAngles), WhlAng/1
  Unary Minus/1 -> YawRate/1
  Wheel to Body Transform/3(zdotWheel) -> Reshape5/1  "Vz"
  VehVel/1 -> Wheel to Body Transform/1(VelVeh)
  r/1 -> Unary Minus/1
  SteerAng/1 -> Wheel Angles/1(SteerAng)
  Wheel to Body Transform/2(ydotWheel) -> Reshape2/1  "Vy"
  Wheel to Body Transform/1(xdotWheel) -> Reshape1/1  "Vx"
  Fz/1 -> Fext/1

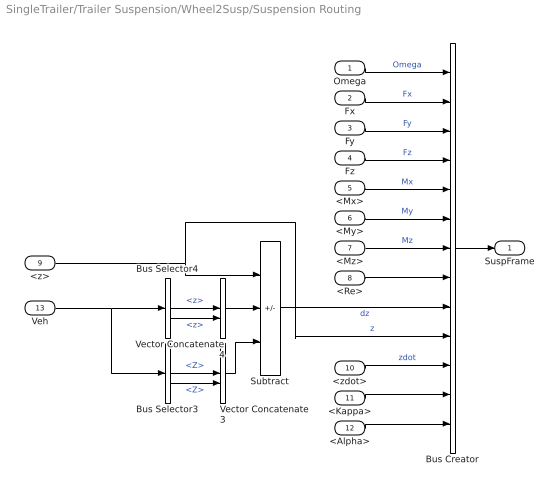
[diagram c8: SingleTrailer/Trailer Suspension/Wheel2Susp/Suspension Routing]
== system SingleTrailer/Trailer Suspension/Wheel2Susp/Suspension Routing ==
  Omega : Inport
  Fx : Inport  Port=2
  Fy : Inport  Port=3
  Fz : Inport  Port=4
  <Mx> : Inport  Port=5
  <My> : Inport  Port=6
  <Mz> : Inport  Port=7
  <Re> : Inport  Port=8
  <z> : Inport  Port=9
  <zdot> : Inport  Port=10
  <Kappa> : Inport  Port=11
  <Alpha> : Inport  Port=12
  Veh : Inport  Port=13
  Bus Creator : BusCreator  Inputs=13
  Bus Selector3 : BusSelector  OutputSignals=InertFrm.FrntAxl.Lft.Disp.Z,InertFrm.FrntAxl.Rght.Disp.Z
  Bus Selector4 : BusSelector  OutputSignals=BdyFrm.FrntAxl.Lft.Disp.z,BdyFrm.FrntAxl.Rght.Disp.z
  Subtract : Sum  Inputs=--+
  Vector Concatenate3 : Concatenate
  Vector Concatenate4 : Concatenate
  SuspFrame : Outport  VectorParamsAs1DForOutWhenUnconnected=off
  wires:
  Bus Selector3/2 -> Vector Concatenate3/2  "<Z>"
  Bus Selector4/2 -> Vector Concatenate4/2  "<z>"
  Vector Concatenate4/1 -> Subtract/2
  Vector Concatenate3/1 -> Subtract/3
  Bus Selector3/1 -> Vector Concatenate3/1  "<Z>"
  Bus Selector4/1 -> Vector Concatenate4/1  "<z>"
  Subtract/1 -> Bus Creator/9  "dz"
  Veh/1 -> Bus Selector4/1, Bus Selector3/1
  <Alpha>/1 -> Bus Creator/13
  <My>/1 -> Bus Creator/6  "My"
  <Mx>/1 -> Bus Creator/5  "Mx"
  <Kappa>/1 -> Bus Creator/12
  Fx/1 -> Bus Creator/2  "Fx"
  Omega/1 -> Bus Creator/1  "Omega"
  Fy/1 -> Bus Creator/3  "Fy"
  Bus Creator/1 -> SuspFrame/1
  <zdot>/1 -> Bus Creator/11  "zdot"
  <Mz>/1 -> Bus Creator/7  "Mz"
  Fz/1 -> Bus Creator/4  "Fz"
  <z>/1 -> Bus Creator/10, Subtract/1  "z"
  <Re>/1 -> Bus Creator/8

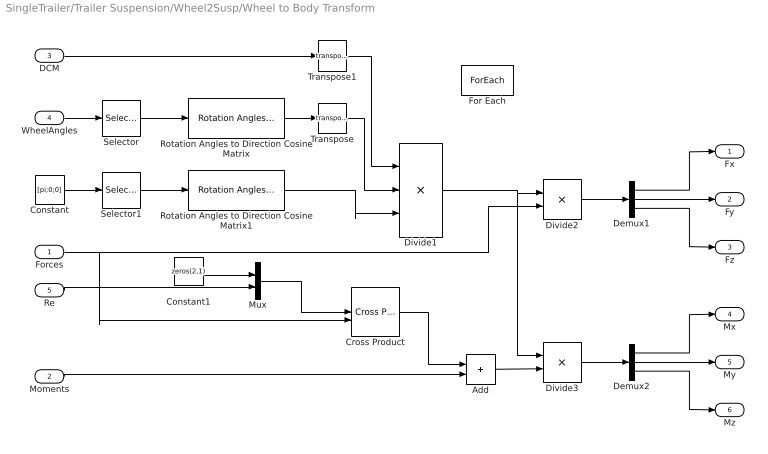
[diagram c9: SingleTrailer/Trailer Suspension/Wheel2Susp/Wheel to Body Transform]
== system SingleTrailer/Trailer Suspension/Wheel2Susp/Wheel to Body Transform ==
  Forces : Inport  PortDimensions=[3,1]  Partition=on  PartitionDimension=2  PartitionWidth=1  PartitionOffset=0
  Moments : Inport  Port=2  PortDimensions=[3,1]  Partition=on  PartitionDimension=2  PartitionWidth=1  PartitionOffset=0
  DCM : Inport  Port=3  Partition=on  PartitionDimension=3  PartitionWidth=1  PartitionOffset=0
  WheelAngles : Inport  Port=4  Partition=on  PartitionDimension=2  PartitionWidth=1  PartitionOffset=0
  Re : Inport  Port=5  Partition=on  PartitionDimension=1  PartitionWidth=1  PartitionOffset=0
  Add : Sum
  Constant : Constant  Value=[pi;0;0]
  Constant1 : Constant  Value=zeros(2,1)
  Cross Product : matrix_library/Cross Product
  Demux1 : Demux  Outputs=3
  Demux2 : Demux  Outputs=3
  Divide1 : Product  Inputs=***  Multiplication=Matrix(*)
  Divide2 : Product  Inputs=**  Multiplication=Matrix(*)
  Divide3 : Product  Inputs=**  Multiplication=Matrix(*)
  For Each : ForEach  DisableCoverage=on
  Mux : Mux  Inputs=2
  Rotation Angles to Direction Cosine Matrix : sharedtransform/Rotation Angles to Direction Cosine Matrix  rotationOrder=ZYX  aMode=2
  Rotation Angles to Direction Cosine Matrix1 : sharedtransform/Rotation Angles to Direction Cosine Matrix  rotationOrder=ZYX  aMode=2
  Selector : Selector  InputPortWidth=3  IndexOptions=Index vector (dialog)  Indices=[3 2 1]  OutputSizes=1
  Selector1 : Selector  InputPortWidth=3  IndexOptions=Index vector (dialog)  Indices=[3 2 1]  OutputSizes=1
  Transpose : Math  Operator=transpose
  Transpose1 : Math  Operator=transpose
  Fx : Outport  ConcatenationDimension=1  VectorParamsAs1DForOutWhenUnconnected=off
  Fy : Outport  Port=2  ConcatenationDimension=1  VectorParamsAs1DForOutWhenUnconnected=off
  Fz : Outport  Port=3  ConcatenationDimension=1  VectorParamsAs1DForOutWhenUnconnected=off
  Mx : Outport  Port=4  ConcatenationDimension=1  VectorParamsAs1DForOutWhenUnconnected=off
  My : Outport  Port=5  ConcatenationDimension=1  VectorParamsAs1DForOutWhenUnconnected=off
  Mz : Outport  Port=6  ConcatenationDimension=1  VectorParamsAs1DForOutWhenUnconnected=off
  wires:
  Demux1/1 -> Fx/1
  Demux1/2 -> Fy/1
  Demux1/3 -> Fz/1
  Rotation Angles to Direction Cosine Matrix/1 -> Transpose/1
  Forces/1 -> Divide2/2, Cross Product/2
  WheelAngles/1 -> Selector/1
  Selector/1 -> Rotation Angles to Direction Cosine Matrix/1
  Rotation Angles to Direction Cosine Matrix1/1 -> Divide1/3
  Selector1/1 -> Rotation Angles to Direction Cosine Matrix1/1
  Constant/1 -> Selector1/1
  Transpose/1 -> Divide1/2
  DCM/1 -> Transpose1/1
  Transpose1/1 -> Divide1/1
  Divide2/1 -> Demux1/1
  Divide3/1 -> Demux2/1
  Divide1/1 -> Divide3/1, Divide2/1
  Moments/1 -> Add/2
  Demux2/3 -> Mz/1
  Demux2/2 -> My/1
  Demux2/1 -> Mx/1
  Add/1 -> Divide3/2
  Cross Product/1 -> Add/1
  Mux/1 -> Cross Product/1
  Re/1 -> Mux/2
  Constant1/1 -> Mux/1

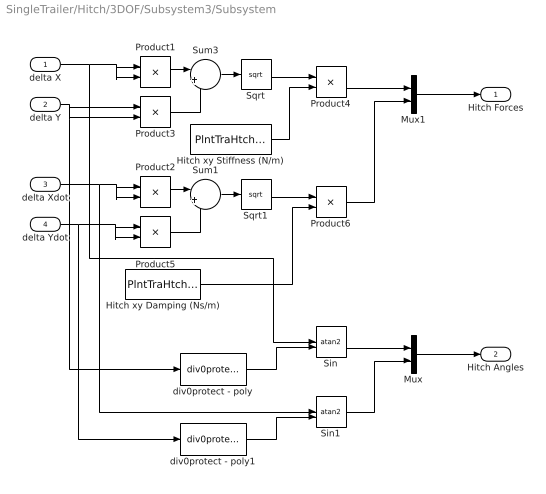
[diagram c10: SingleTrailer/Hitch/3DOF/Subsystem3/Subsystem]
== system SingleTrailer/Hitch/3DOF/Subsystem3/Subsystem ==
  delta X : Inport
  delta Y : Inport  Port=2
  delta Xdot : Inport  Port=3
  delta Ydot : Inport  Port=4
  Hitch xy Damping (Ns/m) : Constant  Value=PlntTraHtchCxy  SampleTime=-1
  Hitch xy Stiffness (N/m) : Constant  Value=PlntTraHtchKxy  SampleTime=-1
  Mux : Mux  Inputs=2
  Mux1 : Mux  Inputs=2
  Product{1..6} (6 alike) : Product
  Sin : Trigonometry  Operator=atan2
  Sin1 : Trigonometry  Operator=atan2
  Sqrt : Sqrt
  Sqrt1 : Sqrt
  Sum1 : Sum  Inputs=|++
  Sum3 : Sum  Inputs=|++
  div0protect - poly : autolibutils/div0protect - poly  thresh=eps  ZeroCross=off  ZeroCross1=off  aMode=2
  div0protect - poly1 : autolibutils/div0protect - poly  thresh=eps  ZeroCross=off  ZeroCross1=off  aMode=2
  Hitch Forces : Outport
  Hitch Angles : Outport  Port=2
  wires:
  div0protect - poly/1 -> Sin/2
  Sin/1 -> Mux/1
  delta X/1 -> Sin/1, Product1/1, Product1/2
  delta Y/1 -> Product3/1, Product3/2, div0protect - poly/1
  Sum3/1 -> Sqrt/1
  Product1/1 -> Sum3/1
  Product3/1 -> Sum3/2
  Sqrt/1 -> Product4/1
  Product4/1 -> Mux1/1
  Hitch xy Stiffness (N/m)/1 -> Product4/2
  Sqrt1/1 -> Product6/1
  Product5/1 -> Sum1/2
  Product2/1 -> Sum1/1
  Sum1/1 -> Sqrt1/1
  delta Xdot/1 -> Sin1/1, Product2/2, Product2/1
  Hitch xy Damping (Ns/m)/1 -> Product6/2
  delta Ydot/1 -> div0protect - poly1/1, Product5/1, Product5/2
  Mux/1 -> Hitch Angles/1
  div0protect - poly1/1 -> Sin1/2
  Sin1/1 -> Mux/2
  Mux1/1 -> Hitch Forces/1
  Product6/1 -> Mux1/2

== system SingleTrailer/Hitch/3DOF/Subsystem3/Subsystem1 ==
  Hitch Forces : Inport
  psi : Inport  Port=2
  Hitch Angles : Inport  Port=3
  Cos : Trigonometry  Operator=cos
  Cos1 : Trigonometry
  Product1 : Product
  Product2 : Product
  Sum : Sum  Inputs=+
  Sum1 : Sum  Inputs=+
  Sum2 : Sum  Inputs=|++
  Fx : Outport
  Fy : Outport  Port=2
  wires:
  Product1/1 -> Sum1/1
  Product2/1 -> Sum/1
  Cos/1 -> Product2/1
  Sum2/1 -> Cos/1, Cos1/1
  psi/1 -> Sum2/2
  Hitch Forces/1 -> Product1/2, Product2/2
  Hitch Angles/1 -> Sum2/1
  Cos1/1 -> Product1/1
  Sum/1 -> Fy/1
  Sum1/1 -> Fx/1

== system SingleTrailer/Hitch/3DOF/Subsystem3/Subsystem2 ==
  Hitch Forces : Inport
  psi : Inport  Port=2
  Hitch Angles : Inport  Port=3
  Cos : Trigonometry  Operator=cos
  Cos1 : Trigonometry
  Gain : Gain  Gain=-1
  Product1 : Product
  Product2 : Product
  Sum : Sum  Inputs=+
  Sum1 : Sum  Inputs=+
  Sum2 : Sum  Inputs=|++
  Fx : Outport
  Fy : Outport  Port=2
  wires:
  Gain/1 -> Product2/2, Product1/2
  Cos1/1 -> Product1/1
  Hitch Angles/1 -> Sum2/1
  Hitch Forces/1 -> Gain/1
  psi/1 -> Sum2/2
  Sum2/1 -> Cos1/1, Cos/1
  Cos/1 -> Product2/1
  Product2/1 -> Sum/1
  Product1/1 -> Sum1/1
  Sum/1 -> Fy/1
  Sum1/1 -> Fx/1

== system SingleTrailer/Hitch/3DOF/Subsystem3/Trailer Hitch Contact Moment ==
  Vehicle Psi : Inport
  Trailer Psi : Inport  Port=2
  Constant : Constant  Value=0  SampleTime=-1
  Hitch Contact Yaw Moment : Lookup_n-D  NumberOfTableDimensions=1  LookupTableObject=''  BreakpointsForDimension1=[-1 -.9 -45*pi/180 0 45*pi/180 .9 1]  BreakpointsForDimension1FirstPoint=10  BreakpointsForDimension2FirstPoint=10  BreakpointsForDimension1Spacing=12  BreakpointsForDimension2Spacing=12  IndexSearchMethod=Linear search  Table=[-1e6 -1e6 0 0 0 1e6 1e6]  ExtrapMethod=Clip  DiagnosticForOutOfRangeInput=Error  UseLastTableValue=on  InternalRulePriority=Speed  RndMeth=Simplest
  Subtract : Sum  Inputs=+-
  Vector Concatenate1 : Concatenate  NumInputs=3
  Mh : Outport
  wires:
  Trailer Psi/1 -> Subtract/2
  Subtract/1 -> Hitch Contact Yaw Moment/1
  Vehicle Psi/1 -> Subtract/1
  Hitch Contact Yaw Moment/1 -> Vector Concatenate1/3
  Constant/1 -> Vector Concatenate1/2, Vector Concatenate1/1
  Vector Concatenate1/1 -> Mh/1

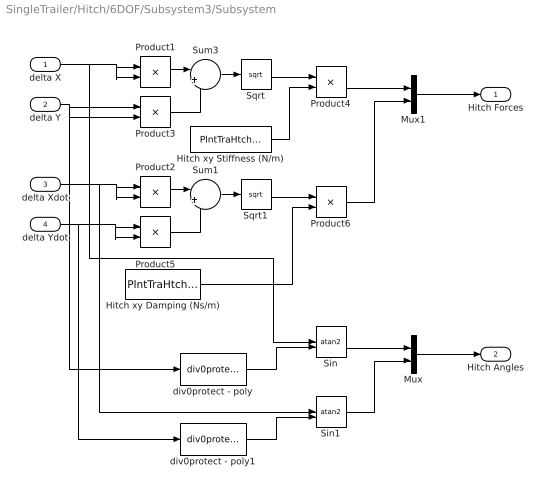
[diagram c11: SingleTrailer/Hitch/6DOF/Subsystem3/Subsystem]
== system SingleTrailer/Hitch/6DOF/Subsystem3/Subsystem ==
  delta X : Inport
  delta Y : Inport  Port=2
  delta Xdot : Inport  Port=3
  delta Ydot : Inport  Port=4
  Hitch xy Damping (Ns/m) : Constant  Value=PlntTraHtchCxy  SampleTime=-1
  Hitch xy Stiffness (N/m) : Constant  Value=PlntTraHtchKxy  SampleTime=-1
  Mux : Mux  Inputs=2
  Mux1 : Mux  Inputs=2
  Product{1..6} (6 alike) : Product
  Sin : Trigonometry  Operator=atan2
  Sin1 : Trigonometry  Operator=atan2
  Sqrt : Sqrt
  Sqrt1 : Sqrt
  Sum1 : Sum  Inputs=|++
  Sum3 : Sum  Inputs=|++
  div0protect - poly : autolibutils/div0protect - poly  thresh=eps  ZeroCross=off  ZeroCross1=off  aMode=2
  div0protect - poly1 : autolibutils/div0protect - poly  thresh=eps  ZeroCross=off  ZeroCross1=off  aMode=2
  Hitch Forces : Outport
  Hitch Angles : Outport  Port=2
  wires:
  div0protect - poly/1 -> Sin/2
  Sin/1 -> Mux/1
  delta X/1 -> Sin/1, Product1/1, Product1/2
  delta Y/1 -> Product3/1, Product3/2, div0protect - poly/1
  Sum3/1 -> Sqrt/1
  Product1/1 -> Sum3/1
  Product3/1 -> Sum3/2
  Sqrt/1 -> Product4/1
  Product4/1 -> Mux1/1
  Hitch xy Stiffness (N/m)/1 -> Product4/2
  Sqrt1/1 -> Product6/1
  Product5/1 -> Sum1/2
  Product2/1 -> Sum1/1
  Sum1/1 -> Sqrt1/1
  delta Xdot/1 -> Sin1/1, Product2/2, Product2/1
  Hitch xy Damping (Ns/m)/1 -> Product6/2
  delta Ydot/1 -> div0protect - poly1/1, Product5/1, Product5/2
  Mux/1 -> Hitch Angles/1
  div0protect - poly1/1 -> Sin1/2
  Sin1/1 -> Mux/2
  Mux1/1 -> Hitch Forces/1
  Product6/1 -> Mux1/2

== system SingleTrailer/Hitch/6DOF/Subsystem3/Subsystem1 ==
  Hitch Forces : Inport
  psi : Inport  Port=2
  Hitch Angles : Inport  Port=3
  Cos : Trigonometry  Operator=cos
  Cos1 : Trigonometry
  Product1 : Product
  Product2 : Product
  Sum : Sum  Inputs=+
  Sum1 : Sum  Inputs=+
  Sum2 : Sum  Inputs=|++
  Fx : Outport
  Fy : Outport  Port=2
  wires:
  Cos1/1 -> Product1/1
  Hitch Angles/1 -> Sum2/1
  Hitch Forces/1 -> Product2/2, Product1/2
  psi/1 -> Sum2/2
  Sum2/1 -> Cos1/1, Cos/1
  Cos/1 -> Product2/1
  Product2/1 -> Sum/1
  Product1/1 -> Sum1/1
  Sum/1 -> Fy/1
  Sum1/1 -> Fx/1

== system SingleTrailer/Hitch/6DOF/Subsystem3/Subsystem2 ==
  Hitch Forces : Inport
  psi : Inport  Port=2
  Hitch Angles : Inport  Port=3
  Cos : Trigonometry  Operator=cos
  Cos1 : Trigonometry
  Gain : Gain  Gain=-1
  Product1 : Product
  Product2 : Product
  Sum : Sum  Inputs=+
  Sum1 : Sum  Inputs=+
  Sum2 : Sum  Inputs=|++
  Fx : Outport
  Fy : Outport  Port=2
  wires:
  Product1/1 -> Sum1/1
  Product2/1 -> Sum/1
  Cos/1 -> Product2/1
  Sum2/1 -> Cos/1, Cos1/1
  psi/1 -> Sum2/2
  Hitch Forces/1 -> Gain/1
  Hitch Angles/1 -> Sum2/1
  Cos1/1 -> Product1/1
  Gain/1 -> Product1/2, Product2/2
  Sum/1 -> Fy/1
  Sum1/1 -> Fx/1

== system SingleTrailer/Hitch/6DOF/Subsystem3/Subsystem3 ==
  Vehicle Z : Inport
  Trailer Z : Inport  Port=2
  Vehicle Zdot : Inport  Port=3
  Trailer Zdot : Inport  Port=4
  Constant8 : Constant  Value=PlntTraHtchF0z  SampleTime=-1
  Gain5 : Gain  Gain=PlntTraHtchKz
  Gain6 : Gain  Gain=PlntTraHtchCz
  Sum1 : Sum  Inputs=|--
  Sum2 : Sum  Inputs=|+-
  Sum3 : Sum  Inputs=|+-
  Sum4 : Sum  Inputs=|+-
  Trailer Fz : Outport
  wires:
  Vehicle Z/1 -> Sum2/2
  Sum4/1 -> Trailer Fz/1
  Gain5/1 -> Sum1/1
  Constant8/1 -> Sum4/2
  Sum1/1 -> Sum4/1
  Gain6/1 -> Sum1/2
  Sum2/1 -> Gain5/1
  Trailer Zdot/1 -> Sum3/1
  Vehicle Zdot/1 -> Sum3/2
  Sum3/1 -> Gain6/1
  Trailer Z/1 -> Sum2/1
